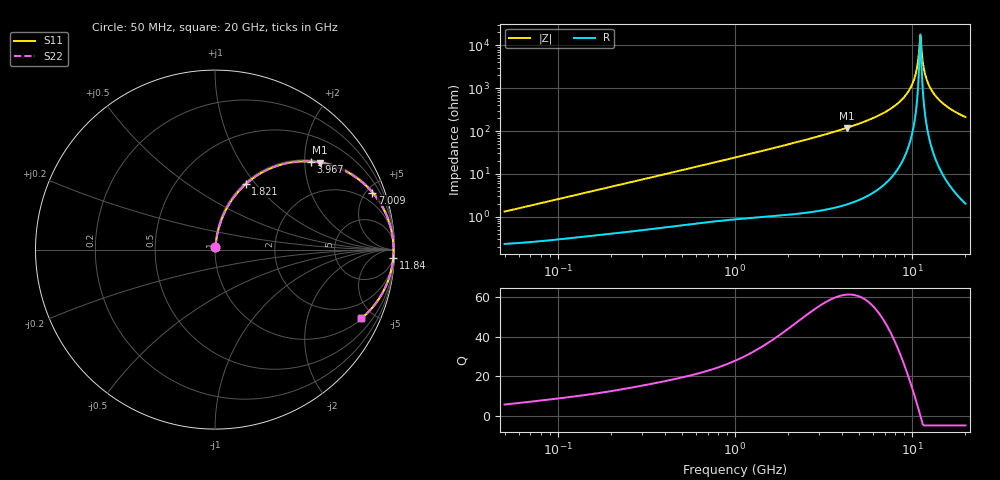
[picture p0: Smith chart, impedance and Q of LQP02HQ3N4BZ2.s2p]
!Murata Part Number: LQP02HQ3N4BZ2
!These Parameters are Measured in Series Mode Connection
!  o--[Z]--o
!Port1  Port2
!  o-------o
!Freq. Start=50[MHz] Stop=20[GHz], 401[Steps]
# Hz S RI R 50
!Freq.(Hz) S11(Real) S11(Imag) S21(Real) S21(Imag) S12(Real) S12(Imag) S22(Real) S22(Imag)
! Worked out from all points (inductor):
!   401 points, 50 MHz to 20 GHz, reference 50 ohm
!   read as one part in series: L = 4.11 nH near 51.52 MHz
!   highest Q = 61.3 at 4.276 GHz (marker M1), where L = 4.41 nH
!   self-resonance near 10.99 GHz
!   S11 on the Smith chart (normalised r, x): 50 MHz: 1.00, +0.03; 1.821 GHz: 1.02, +0.89; 3.967 GHz: 1.04, +2.15; 7.009 GHz: 1.12, +5.48; 11.84 GHz: 6, -42; 20 GHz: 1.04, -4.24
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5e7  0.00248 0.0129  0.9975 -0.0129  0.9975 -0.0129  0.00248 0.0129
1.364002e8  0.00454 0.0342  0.9955 -0.0342  0.9955 -0.0342  0.00454 0.0342
3.721004e8  0.0135 0.0894  0.9865 -0.0894  0.9865 -0.0894  0.0135 0.0894
1e9  0.062 0.2239  0.938 -0.2239  0.938 -0.2239  0.062 0.2239
1.820564e9  0.1702 0.3639  0.8298 -0.3639  0.8298 -0.3639  0.1702 0.3639
2.728004e9  0.3232 0.4584  0.6768 -0.4584  0.6768 -0.4584  0.3232 0.4584
3.967106e9  0.5346 0.4907  0.4654 -0.4907  0.4654 -0.4907  0.5346 0.4907
4.275624e9  0.5823 0.4851  0.4177 -0.4851  0.4177 -0.4851  0.5823 0.4851
7.009217e9  0.8772 0.3178  0.1228 -0.3178  0.1228 -0.3178  0.8772 0.3178
7.442007e9  0.9042 0.2829  0.0958 -0.2829  0.0958 -0.2829  0.9042 0.2829
8.774992e9  0.9618 0.175  0.0382 -0.175  0.0382 -0.175  0.9618 0.175
9.745021e9  0.984 0.0997  0.016 -0.0997  0.016 -0.0997  0.984 0.0997
1.034674e10  0.9912 0.0553  0.00876 -0.0553  0.00876 -0.0553  0.9912 0.0553
1.066139e10  0.9933 0.0328  0.00667 -0.0328  0.00667 -0.0328  0.9933 0.0328
1.082228e10  0.994 0.0216  0.00601 -0.0216  0.00601 -0.0216  0.994 0.0216
1.115139e10  0.9945 -0.000989  0.00545 0.000989  0.00545 0.000989  0.9945 -0.000989
1.149051e10  0.9941 -0.0235  0.00593 0.0235  0.00593 0.0235  0.9941 -0.0235
1.183995e10  0.9926 -0.046  0.00743 0.046  0.00743 0.046  0.9926 -0.046
1.257102e10  0.9865 -0.0907  0.0135 0.0907  0.0135 0.0907  0.9865 -0.0907
1.396067e10  0.9663 -0.1668  0.0337 0.1668  0.0337 0.1668  0.9663 -0.1668
1.646126e10  0.9113 -0.2767  0.0887 0.2767  0.0887 0.2767  0.9113 -0.2767
2e10  0.8157 -0.383  0.1843 0.383  0.1843 0.383  0.8157 -0.383
